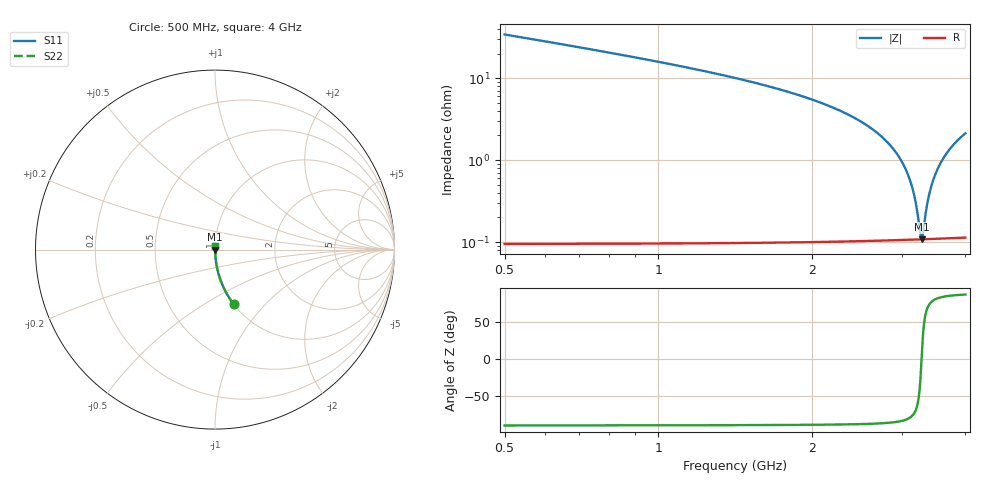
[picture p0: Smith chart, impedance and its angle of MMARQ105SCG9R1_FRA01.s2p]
! MMARQ105SCG9R1_FRA01  S-PARAMETER MODEL  ( General Type )
! Model Generated by TAIYO YUDEN Corporation (http://www.ty-top.com)
! Version 1.0
! TAIYO YUDEN Control No. 200326
! Copyright(c) 2020 TAIYO YUDEN CO.,LTD. All Rights Reserved.
! Product Description (link to TY-COMPAS)
! https://ds.yuden.co.jp/TYCOMPAS/or/detail?pn=MMARQ105SCG9R1CFRA01&u=M
! Products Name : Multilayer Ceramic Capacitors
! Characteristics :
!  Capacitance : 9.1 pF , Rated Voltage : 250V , TCC : CG / C0G
!  Case Size : 1.0 x 0.5 / 0.039 x 0.02 [mm/inch] , Thickness : 0.5 / 0.02 [mm/inch]
!  (Conditions: Temperature = 25 degC , DC Bias Current/Voltage = 0A / 0V)
! External Node Assignments :
!  1  o---| |---o  2
! GND o---------o GND
! Frequency Range : 500MHz  -  4GHz  [ 401 STEP ]
# MHz S RI R 50
! Freq[MHz].  S11 Real  S11 Imag  S21 Real  S21 Imag  S12 Real  S12 Imag  S22 Real  S22 Imag
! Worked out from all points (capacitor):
!   401 points, 500 MHz to 4 GHz, reference 50 ohm
!   read as one part in series: C = 9.09 pF near 517.5 MHz
!   lowest |Z| = 108 mohm at 3.283 GHz (marker M1)
!   series resonance near 3.282 GHz, so ESL is about 260 pH
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500  0.1053 -0.3056  0.8947 0.3056  0.8947 0.3056  0.1053 -0.3056
762.5  0.0459 -0.207  0.9541 0.207  0.9541 0.207  0.0459 -0.207
1086.25  0.0211 -0.1403  0.9789 0.1403  0.9789 0.1403  0.0211 -0.1403
1672.5  0.00693 -0.0768  0.9931 0.0768  0.9931 0.0768  0.00693 -0.0768
2250  0.0027 -0.0411  0.9973 0.0411  0.9973 0.0411  0.0027 -0.0411
2582.5  0.00169 -0.0257  0.9983 0.0257  0.9983 0.0257  0.00169 -0.0257
2836.25  0.00129 -0.0156  0.9987 0.0156  0.9987 0.0156  0.00129 -0.0156
3002.5  0.00115 -0.00949  0.9989 0.00949  0.9989 0.00949  0.00115 -0.00949
3063.75  0.00112 -0.00734  0.9989 0.00734  0.9989 0.00734  0.00112 -0.00734
3116.25  0.0011 -0.00553  0.9989 0.00553  0.9989 0.00553  0.0011 -0.00553
3186.25  0.00108 -0.00316  0.9989 0.00316  0.9989 0.00316  0.00108 -0.00316
3212.5  0.00108 -0.00229  0.9989 0.00229  0.9989 0.00229  0.00108 -0.00229
3265  0.00108 -0.000568  0.9989 0.000568  0.9989 0.000568  0.00108 -0.000568
3282.5  0.00108 4.8e-08  0.9989 -4.8e-08  0.9989 -4.8e-08  0.00108 4.8e-08
3300  0.00108 0.000565  0.9989 -0.000565  0.9989 -0.000565  0.00108 0.000565
3343.75  0.00109 0.00197  0.9989 -0.00197  0.9989 -0.00197  0.00109 0.00197
3370  0.00109 0.0028  0.9989 -0.0028  0.9989 -0.0028  0.00109 0.0028
3422.5  0.00111 0.00444  0.9989 -0.00444  0.9989 -0.00444  0.00111 0.00444
3518.75  0.00115 0.00739  0.9989 -0.00739  0.9989 -0.00739  0.00115 0.00739
3641.25  0.00123 0.011  0.9988 -0.011  0.9988 -0.011  0.00123 0.011
3807.5  0.00137 0.0158  0.9986 -0.0158  0.9986 -0.0158  0.00137 0.0158
4000  0.00158 0.0211  0.9984 -0.0211  0.9984 -0.0211  0.00158 0.0211
